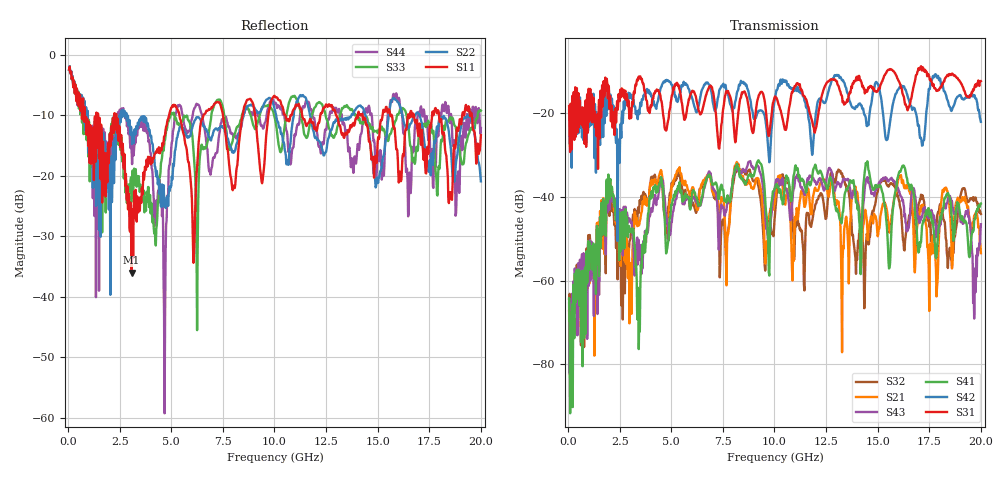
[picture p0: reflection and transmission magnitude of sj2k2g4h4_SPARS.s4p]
! FILE: E:\users\goganessyan\GBX_Backplane\FR408_backplane\1m_INBOUND_NEXT\sj2k2g4h4_SPARS.s4p
# MHZ S RI R 50.00
! FREQ  S11  S12  S13  S14
!  S21  S22  S23  S24
!  S31  S32  S33  S34
!  S41  S42  S43  S44
!  REAL  IMAG  REAL  IMAG  REAL  IMAG  REAL  IMAG
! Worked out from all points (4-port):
!   799 points, 50 MHz to 20 GHz, reference 50 ohm
!   strongest paths, dB at 50 MHz, 5.025 GHz, 10.03 GHz, 15.03 GHz, 20 GHz:
!     S31: -18.3, -15.8, -16.0, -14.5, -12.4
!     S42: -19.3, -13.3, -16.4, -13.2, -22.1
!     S41: -64.3, -41.9, -37.9, -37.5, -41.6
!     S43: -65.4, -46.0, -37.5, -37.4, -46.6
!     S21: -67.3, -37.3, -40.8, -49.0, -53.4
!     S32: -64.3, -36.6, -44.2, -38.1, -44.1
!   lowest |S11| = -36.0 dB at 3.075 GHz (marker M1), VSWR 1.03, Z = 51 + j1.22 ohm
!   |S11| at or under -10 dB: 2.328 GHz to 4.889 GHz (2.561 GHz wide, 71 % of centre); 5.393 GHz to 6.562 GHz (1.168 GHz wide, 19.5 % of centre); 17.97 GHz to 19.1 GHz (1.123 GHz wide, 6.06 % of centre)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
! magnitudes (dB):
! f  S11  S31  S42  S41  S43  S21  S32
! 50 MHz  -2.4  -18.3  -19.3  -64.3  -65.4  -67.3  -64.3
! 1.95 GHz  -14.6  -13.4  -14.8  -34.7  -36.1  -35.5  -37.5
! 3.075 GHz  -36.0  -19.5  -15.7  -47.6  -46.0  -67.9  -47.6
! 4.7 GHz  -13.2  -24.0  -12.2  -47.0  -41.5  -44.4  -45.4
! 5.325 GHz  -9.2  -13.5  -17.0  -37.4  -38.4  -33.4  -35.0
! 8.2 GHz  -18.2  -22.2  -14.8  -32.3  -33.1  -32.0  -33.9
! 20 GHz  -13.3  -12.4  -22.1  -41.6  -46.6  -53.4  -44.1
